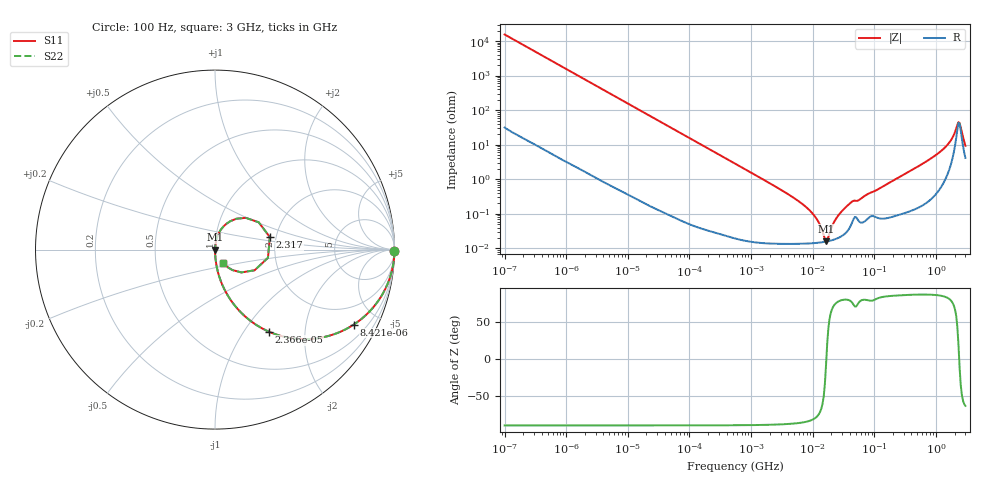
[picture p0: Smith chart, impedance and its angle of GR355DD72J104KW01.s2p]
!Murata Part Number: GR355DD72J104KW01
!These Parameters are Measured in Series Mode Connection
!Data Generated on Jan 08, 2026
!  o--ll--o
!Port1  Port2
!  o------o
!Operation Temp=25[degC], DC Bias Voltage=0[V]
!Freq. Start=100[Hz] Stop=3[GHz] 401[Steps]
# Hz S RI R 50
!Freq.(Hz) S11(Real) S11(Imag) S21(Real) S21(Imag) S12(Real) S12(Imag) S22(Real) S22(Imag)
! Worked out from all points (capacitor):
!   401 points, 100 Hz to 3 GHz, reference 50 ohm
!   read as one part in series: C = 103 nF near 109 Hz
!   lowest |Z| = 16 mohm at 16.42 MHz (marker M1)
!   series resonance near 16.65 MHz, so ESL is about 890 pH
!   S11 on the Smith chart (normalised r, x): 100 Hz: open; 8.421 kHz: 1.01, -3.69; 23.66 kHz: 1.00, -1.32; 2.317 GHz: 1.85, +0.29; 3 GHz: 1.08, -0.17
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100  0.9999 -0.00647  5.51e-05 0.00647  5.51e-05 0.00647  0.9999 -0.00647
1788  0.9866 -0.1138  0.0134 0.1138  0.0134 0.1138  0.9866 -0.1138
4415  0.9246 -0.2629  0.0754 0.2629  0.0754 0.2629  0.9246 -0.2629
8421  0.7724 -0.4182  0.2276 0.4182  0.2276 0.4182  0.7724 -0.4182
23658  0.3023 -0.458  0.6977 0.458  0.6977 0.458  0.3023 -0.458
31977  0.1921 -0.3927  0.8079 0.3927  0.8079 0.3927  0.1921 -0.3927
116311  0.0181 -0.1316  0.9819 0.1316  0.9819 0.1316  0.0181 -0.1316
547723  0.00101 -0.0285  0.999 0.0285  0.999 0.0285  0.00101 -0.0285
4323298  0.000147 -0.00338  0.9999 0.00338  0.9999 0.00338  0.000147 -0.00338
9794414  0.000142 -0.00105  0.9999 0.00105  0.9999 0.00105  0.000142 -0.00105
1.214626e7  0.000147 -0.000604  0.9999 0.000604  0.9999 0.000604  0.000147 -0.000604
1.641694e7  0.000158 -2.58e-05  0.9998 2.58e-05  0.9998 2.58e-05  0.000158 -2.58e-05
1.789277e7  0.000163 0.000137  0.9998 -0.000137  0.9998 -0.000137  0.000163 0.000137
2.418395e7  0.000192 0.000728  0.9998 -0.000728  0.9998 -0.000728  0.000192 0.000728
3.882828e7  0.000374 0.00188  0.9996 -0.00188  0.9996 -0.00188  0.000374 0.00188
1.751444e8  0.000841 0.00792  0.9992 -0.00792  0.9992 -0.00792  0.000841 0.00792
1.114774e9  0.00812 0.0576  0.9919 -0.0576  0.9919 -0.0576  0.00812 0.0576
1.573002e9  0.0253 0.0992  0.9747 -0.0992  0.9747 -0.0992  0.0253 0.0992
2.036508e9  0.1194 0.1721  0.8806 -0.1721  0.8806 -0.1721  0.1194 0.1721
2.317205e9  0.3055 0.0699  0.6945 -0.0699  0.6945 -0.0699  0.3055 0.0699
2.636591e9  0.1465 -0.1271  0.8535 0.1271  0.8535 0.1271  0.1465 -0.1271
3e9  0.046 -0.0763  0.954 0.0763  0.954 0.0763  0.046 -0.0763
